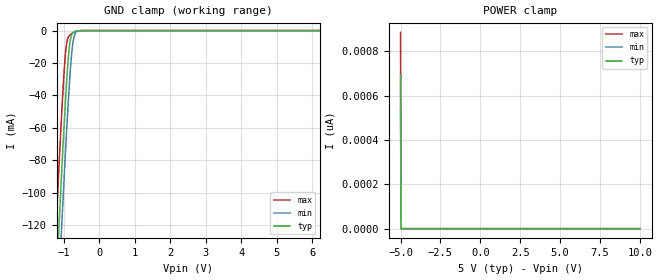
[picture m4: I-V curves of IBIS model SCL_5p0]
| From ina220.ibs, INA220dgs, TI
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|   Model
[Model]   SCL_5p0
Model_type   Input
Vinl = 1.5
Vinh = 3.5
|   typ   min   max
C_comp   1.1266090e-12 9.9319810e-13 1.2181950e-12
[Voltage Range]   5   4.5   5.5
[Temperature Range]   27   85   -40
[Power Clamp Reference]   5   4.5   5.5
[GND Clamp Reference]   -0   -0   -0
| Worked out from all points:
|   GND clamp passes 1 mA (typ) near -0.72 V on its own axis
[GND Clamp]
|   Voltage   I(typ)   I(min)   I(max)
-5V       -2.019A    -2.05A     -1.986A
-1.25V    -175.5mA   -209.9mA   -138.2mA
-1.145V   -127.2mA   -161.5mA   -90.2mA
-1.13V    -120.5mA   -154.6mA   -83.53mA
-1.07V    -93.79mA   -127.6mA   -57.58mA
-1.055V   -87.25mA   -121mA     -51.35mA
-950mV    -44mA      -75.77mA   -14.53mA
-860mV    -14.64mA   -40.6mA    -3.754mA
-815mV    -6.104mA   -25.5mA    -2.622mA
-755mV    -1.796mA   -10.25mA   -1.584mA
-665mV    -405.7uA   -1.312mA   -516.6uA
9.985V    0A         0A         0A
[POWER Clamp]
|   Voltage   I(typ)   I(min)   I(max)
-5V       693.1pA    550.8pA    885.1pA
-4.97V    0A         0A         0A
-4.955V   0A         0A         0A
9.985V    0A         0A         0A
